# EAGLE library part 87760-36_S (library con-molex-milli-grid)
HEADER
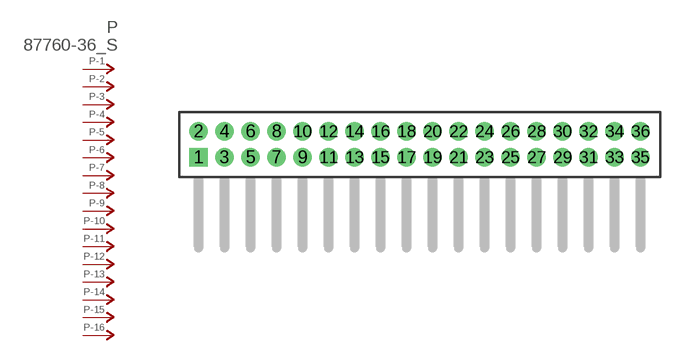
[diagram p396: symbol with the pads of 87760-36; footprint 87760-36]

Designator prefix P; gates -1=P-NV -2=P-N -3=P-N -4=P-N -5=P-N -6=P-N -7=P-N -8=P-N -9=P-N -10=P-N -11=P-N -12=P-N -13=P-N -14=P-N -15=P-N -16=P-N -17=P-N -18=P-N -19=P-N -20=P-N -21=P-N -22=P-N -23=P-N -24=P-N -25=P-N -26=P-N -27=P-N -28=P-N -29=P-N -30=P-N -31=P-N -32=P-N -33=P-N -34=P-N -35=P-N -36=P-N

## 87760-36_S  [87760-36]
1  -1:P  pas
2  -2:P  pas
3  -3:P  pas
4  -4:P  pas
5  -5:P  pas
6  -6:P  pas
7  -7:P  pas
8  -8:P  pas
9  -9:P  pas
10  -10:P  pas
11  -11:P  pas
12  -12:P  pas
13  -13:P  pas
14  -14:P  pas
15  -15:P  pas
16  -16:P  pas
17  -17:P  pas
18  -18:P  pas
19  -19:P  pas
20  -20:P  pas
21  -21:P  pas
22  -22:P  pas
23  -23:P  pas
24  -24:P  pas
25  -25:P  pas
26  -26:P  pas
27  -27:P  pas
28  -28:P  pas
29  -29:P  pas
30  -30:P  pas
31  -31:P  pas
32  -32:P  pas
33  -33:P  pas
34  -34:P  pas
35  -35:P  pas
36  -36:P  pas

## Footprint 87760-36 (pad centres in mm)
HEADER Dual Row, Right Angle
drill 0.914 square: 1 -17,-1
drill 0.914: 2 -17,1; 3 -15,-1; 4 -15,1; 5 -13,-1; 6 -13,1; 7 -11,-1; 8 -11,1; 9 -9,-1; 10 -9,1; 11 -7,-1; 12 -7,1; 13 -5,-1; 14 -5,1; 15 -3,-1; 16 -3,1; 17 -1,-1; 18 -1,1; 19 1,-1; 20 1,1; 21 3,-1; 22 3,1; 23 5,-1; 24 5,1; 25 7,-1; 26 7,1; 27 9,-1; 28 9,1; 29 11,-1; 30 11,1; 31 13,-1; 32 13,1; 33 15,-1; 34 15,1; 35 17,-1; 36 17,1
